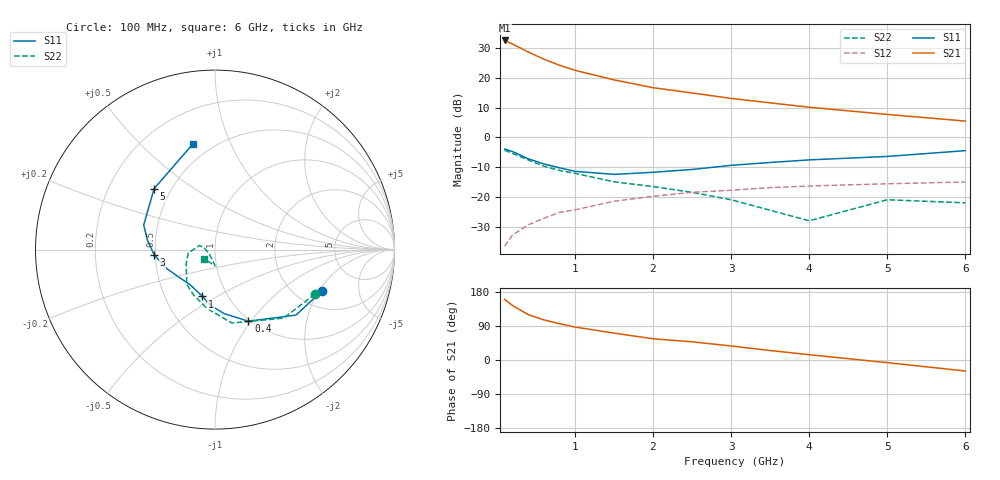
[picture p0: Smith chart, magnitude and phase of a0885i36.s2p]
!  MSA-0885 S AND NOISE PARAMETERS
!  Id=36mA  LAST UPDATED 07-27-92
# ghz s ma r 50
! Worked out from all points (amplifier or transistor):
!   14 points, 100 MHz to 6 GHz, reference 50 ohm
!   highest |S21| = 32.5 dB at 100 MHz (marker M1)
!   |S21| within 3 dB of that: start of sweep to 337 MHz
!   unconditionally stable (mu >= 1): 2.523 GHz to end of sweep
!   at 400 MHz: K = 0.69, MSG = 29.0 dB, |S12| = -29.4 dB
!   at 2 GHz: K = 0.98, MSG = 18.2 dB, |S12| = -19.7 dB
!   at 6 GHz: K = 1.07, MAG = 8.6 dB, |S12| = -14.9 dB
!   lowest NFmin = 2.70 dB at 100 MHz
!   S11 on the Smith chart (normalised r, x): 100 MHz: 2.75, -2.14; 400 MHz: 0.98, -0.97; 1 GHz: 0.76, -0.43; 3 GHz: 0.49, -0.03; 5 GHz: 0.40, +0.36; 6 GHz: 0.40, +0.73
0.1  0.64 -21.0  42.29 160.0  0.015 40.0  0.61 -24.0
0.2  0.58 -39.0  36.89 144.0  0.023 50.0  0.54 -45.0
0.4  0.44 -65.0  27.2 120.0  0.034 54.0  0.42 -77.0
0.6  0.36 -82.0  20.57 106.0  0.044 53.0  0.33 -98.0
0.8  0.31 -95.0  16.31 96.0  0.055 53.0  0.28 -115.0
1  0.27 -105.0  13.36 87.0  0.061 51.0  0.25 -129.0
1.5  0.24 -125.0  9.24 71.0  0.085 50.0  0.18 -153.0
2  0.26 -147.0  6.82 56.0  0.103 47.0  0.15 -173.0
2.5  0.29 -159.0  5.57 48.0  0.12 44.0  0.12 180.0
3  0.34 -175.0  4.51 37.0  0.13 42.0  0.09 165.0
3.5  0.38 172.0  3.8 25.0  0.144 37.0  0.06 172.0
4  0.42 161.0  3.21 14.0  0.153 33.0  0.04 -139.0
5  0.48 135.0  2.43 -7.0  0.167 24.0  0.09 -90.0
6  0.6 102.0  1.88 -29.0  0.179 17.0  0.08 -140.0
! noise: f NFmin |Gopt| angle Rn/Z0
0.1  2.7  0.36  1  0.63
0.5  2.8  0.35  5  0.63
1  3  0.33  10  0.63
2  3.6  0.23  16  0.62
